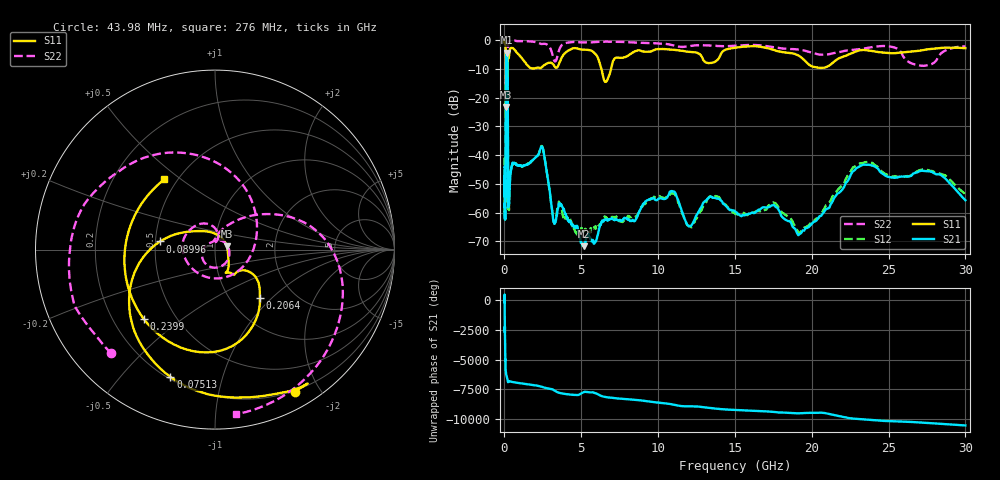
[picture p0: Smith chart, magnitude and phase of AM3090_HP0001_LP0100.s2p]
! Date/Time: Thu, Feb 28, 2019 1:54 PM
! Network Analyzer: Agilent Technologies E8364B Rev: A.07.50.67
! Sweep from 0.010 to 30.000 GHz, 1601 Points, Sweep Type: LOG
! Power Supply: 5.023 V, 0.002 A
# Hz S DB R 50
!freq MagS11 AngS11 MagS21 AngS21 MagS12 AngS12 MagS22 AngS22
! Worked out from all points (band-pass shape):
!   1601 points, 10 MHz to 30 GHz, reference 50 ohm
!   highest |S21| = -4.39 dB at 141.8 MHz (marker M1); lowest = -71.7 dB at 5.154 GHz (marker M2)
!   |S21| within 3 dB of the highest: 99.42 MHz to 196.3 MHz (96.86 MHz wide, 65.5 % of centre)
!   lowest |S11| = -23.3 dB at 98.44 MHz (marker M3), VSWR 1.15, Z = 57 + j2.23 ohm
!   |S11| at or under -10 dB: 89.83 MHz to 199.6 MHz (109.7 MHz wide, 75.8 % of centre); 6.309 GHz to 6.936 GHz (627.7 MHz wide, 9.48 % of centre)
!   |S22| runs from -27.5 to -0.1 dB; largest |S21 - S12| = 0.011
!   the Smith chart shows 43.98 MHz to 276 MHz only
!   S11 on the Smith chart (normalised r, x): 43.98 MHz: 0.19, -1.70; 75.13 MHz: 0.21, -0.69; 89.96 MHz: 0.53, +0.05; 206.4 MHz: 1.36, -0.85; 239.9 MHz: 0.33, -0.37; 276 MHz: 0.43, +0.44
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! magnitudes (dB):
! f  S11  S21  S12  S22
! 10 MHz  -0.3  -44.1  -40.7  -0.5
! 38.04 MHz  -0.5  -61.5  -61.5  -1.4
! 43.98 MHz  -0.8  -60.1  -58.7  -1.7
! 75.13 MHz  -2.5  -47.1  -44.7  -4.6
! 89.96 MHz  -10.2  -15.3  -15.3  -15.7
! 98.44 MHz  -23.3  -7.7  -7.7  -14.7
! 141.8 MHz  -15.6  -4.4  -4.3  -22.9
! 144.7 MHz  -15.5  -4.4  -4.3  -22.1
! 185.8 MHz  -13.8  -5.9  -5.9  -26.9
! 206.4 MHz  -8.7  -10.9  -10.9  -13.6
! 239.9 MHz  -5.1  -54.2  -52.2  -1.7
! 276 MHz  -6.3  -56.6  -57.7  -0.7
! 550.5 MHz  -2.9  -42.7  -43.1  -0.2
! 2.084 GHz  -9.7  -40.5  -40.5  -0.8
! 2.507 GHz  -9.1  -37.9  -37.8  -1.3
! 3.236 GHz  -9.0  -63.8  -63.7  -7.1
! 5.154 GHz  -3.4  -71.7  -66.8  -0.8
! 7.926 GHz  -5.8  -61.9  -62.1  -0.7
! 10.81 GHz  -3.3  -52.6  -53.5  -1.6
! 19.61 GHz  -7.5  -65.4  -65.1  -3.8
! 23.48 GHz  -3.5  -43.3  -42.5  -2.9
! 30 GHz  -2.8  -55.7  -53.6  -2.2
